(* Logix 5000 AddOnInstructionDefinition export Banner_S4B_PD_v5; software revision 33.00 *)

TYPE Banner_S4B_PDI_Host_Guest :
STRUCT
   Reduced_Resolution_Enabled : SINT;   // 0=false, 1=true
   Status : SINT;   // 0=clear, 1=weak beam, 2=blocked
   Indicator_State : SINT;   // 0=Enabled, 1=Override, 2=Dipswitch Disabled
   Measurement : INT;   // 0 to 180
   First_Channel_Blocked : INT;   // 0 to 180
   Number_Channels_Blocked : INT;   // 0 to 180
   Zone_1_Status : SINT;   // 0=clear, 1=weak beam, 2=blocked
   Zone_2_Status : SINT;   // 0=clear, 1=weak beam, 2=blocked
   Zone_3_Status : SINT;   // 0=clear, 1=weak beam, 2=blocked
END_STRUCT
END_TYPE

TYPE Banner_S4B_PDI_v5 :
STRUCT
   OSSD_Status : SINT;   // 0=Off, 1=On
   Weak_Beam_Flag : SINT;   // 0=Maintenance flag not active, 1=Maintenance flag active
   Cascaded_Units : SINT;   // 0=Standalone, 1=1 cascaded unit, 2=2 cascaded units, 3=3 cascaded units
   Configurable_IO_Pin_State : SINT;   // 0=Off, 1=On
   Fixed_Blanking_Enabled : SINT;   // 0=false, 1=true
   Vibration_Tolerance_Enabled : SINT;   // 0=false, 1=true
   Fault_Lockout : SINT;   // 0=false, 1=true
   Diagnostic_Error_Cocde : SINT;   // 0 to 255
   Host : Banner_S4B_PDI_Host_Guest;
   Guest_1 : Banner_S4B_PDI_Host_Guest;
   Guest_2 : Banner_S4B_PDI_Host_Guest;
   Guest_3 : Banner_S4B_PDI_Host_Guest;
END_STRUCT
END_TYPE

TYPE Banner_S4B_PDIO_v5 :   // UDT that records the converted prcoess data.
STRUCT
   PDI : Banner_S4B_PDI_v5;
   PDO : Banner_S4B_PDO_v5;
   PDO_DT : SINT[4];
   PDI_DT : SINT[20];
END_STRUCT
END_TYPE

TYPE Banner_S4B_PDO_v5 :
STRUCT
   Override_Indicator_State_Host : SINT;   // 0=Standard Operation, 1 to 9 = Override 1 to 9
   Override_Indicator_State_Guest_1 : SINT;   // 0=Standard Operation, 1 to 9 = Override 1 to 9
   Override_Indicator_State_Guest_2 : SINT;   // 0=Standard Operation, 1 to 9 = Override 1 to 9
   Override_Indicator_State_Guest_3 : SINT;   // 0=Standard Operation, 1 to 9 = Override 1 to 9
END_STRUCT
END_TYPE

ADD_ON_INSTRUCTION Banner_S4B_PD_v5   (* revision 5.0, vendor Banner Engineering *)
// Takes the raw SINT information and converts that data into actual information.
VAR_IN_OUT
   PD : Banner_S4B_PDIO_v5; {required}
END_VAR
VAR_INPUT
   Byte_Swap : BOOL; {required}
END_VAR
VAR
   PDO_Temp : SINT[4]; {access None}
   PDI_Temp : SINT[20]; {access None}
END_VAR

ROUTINE Logic   (* ladder *)
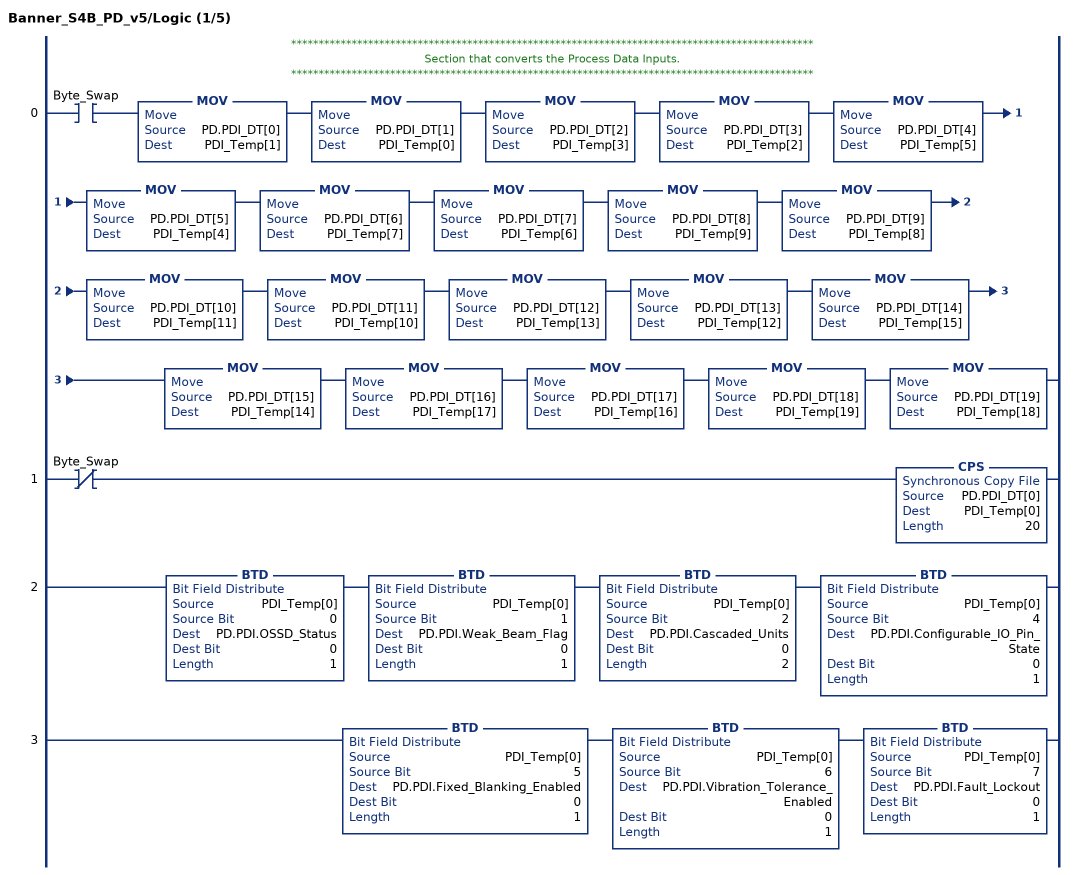
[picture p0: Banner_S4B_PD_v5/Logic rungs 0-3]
   // ***********************************************************************************************
   // Section that converts the Process Data Inputs.
   // ***********************************************************************************************
   0: XIC(Byte_Swap)MOV(PD.PDI_DT[0],PDI_Temp[1])MOV(PD.PDI_DT[1],PDI_Temp[0])MOV(PD.PDI_DT[2],PDI_Temp[3])MOV(PD.PDI_DT[3],PDI_Temp[2])MOV(PD.PDI_DT[4],PDI_Temp[5])MOV(PD.PDI_DT[5],PDI_Temp[4])MOV(PD.PDI_DT[6],PDI_Temp[7])MOV(PD.PDI_DT[7],PDI_Temp[6])MOV(PD.PDI_DT[8],PDI_Temp[9])MOV(PD.PDI_DT[9],PDI_Temp[8])MOV(PD.PDI_DT[10],PDI_Temp[11])MOV(PD.PDI_DT[11],PDI_Temp[10])MOV(PD.PDI_DT[12],PDI_Temp[13])MOV(PD.PDI_DT[13],PDI_Temp[12])MOV(PD.PDI_DT[14],PDI_Temp[15])MOV(PD.PDI_DT[15],PDI_Temp[14])MOV(PD.PDI_DT[16],PDI_Temp[17])MOV(PD.PDI_DT[17],PDI_Temp[16])MOV(PD.PDI_DT[18],PDI_Temp[19])MOV(PD.PDI_DT[19],PDI_Temp[18]);
   1: XIO(Byte_Swap)CPS(PD.PDI_DT[0],PDI_Temp[0],20);
   2: BTD(PDI_Temp[0],0,PD.PDI.OSSD_Status,0,1)BTD(PDI_Temp[0],1,PD.PDI.Weak_Beam_Flag,0,1)BTD(PDI_Temp[0],2,PD.PDI.Cascaded_Units,0,2)BTD(PDI_Temp[0],4,PD.PDI.Configurable_IO_Pin_State,0,1);
   3: BTD(PDI_Temp[0],5,PD.PDI.Fixed_Blanking_Enabled,0,1)BTD(PDI_Temp[0],6,PD.PDI.Vibration_Tolerance_Enabled,0,1)BTD(PDI_Temp[0],7,PD.PDI.Fault_Lockout,0,1);
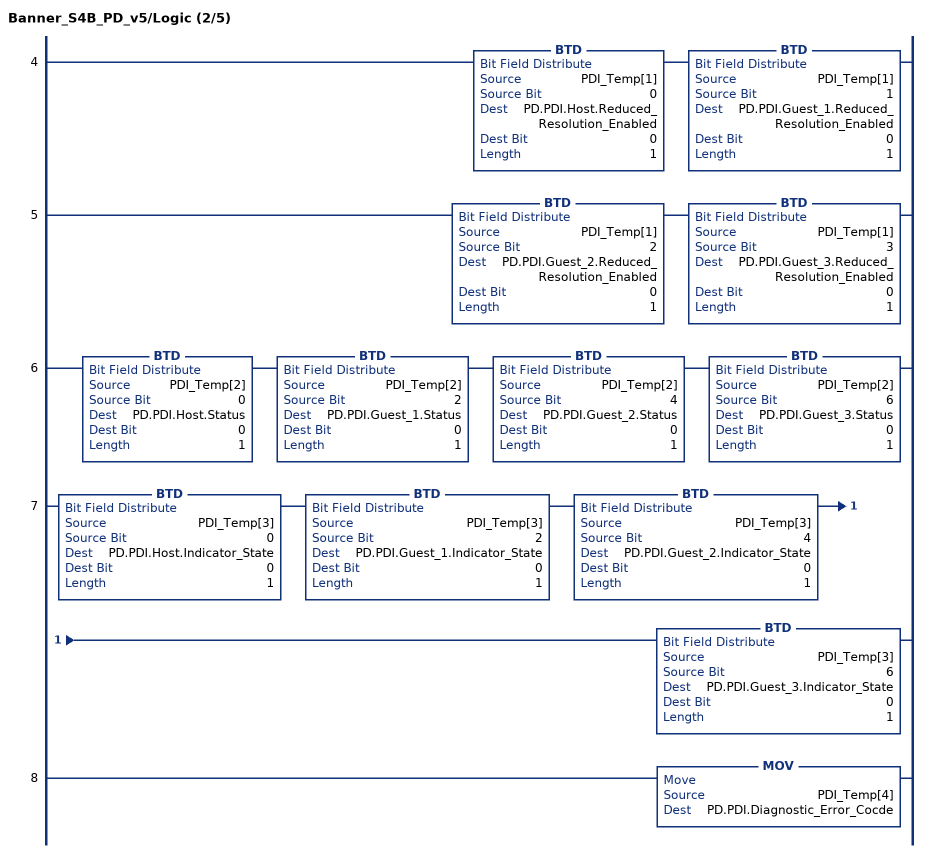
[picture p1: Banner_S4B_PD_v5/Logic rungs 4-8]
   4: BTD(PDI_Temp[1],0,PD.PDI.Host.Reduced_Resolution_Enabled,0,1)BTD(PDI_Temp[1],1,PD.PDI.Guest_1.Reduced_Resolution_Enabled,0,1);
   5: BTD(PDI_Temp[1],2,PD.PDI.Guest_2.Reduced_Resolution_Enabled,0,1)BTD(PDI_Temp[1],3,PD.PDI.Guest_3.Reduced_Resolution_Enabled,0,1);
   6: BTD(PDI_Temp[2],0,PD.PDI.Host.Status,0,1)BTD(PDI_Temp[2],2,PD.PDI.Guest_1.Status,0,1)BTD(PDI_Temp[2],4,PD.PDI.Guest_2.Status,0,1)BTD(PDI_Temp[2],6,PD.PDI.Guest_3.Status,0,1);
   7: BTD(PDI_Temp[3],0,PD.PDI.Host.Indicator_State,0,1)BTD(PDI_Temp[3],2,PD.PDI.Guest_1.Indicator_State,0,1)BTD(PDI_Temp[3],4,PD.PDI.Guest_2.Indicator_State,0,1)BTD(PDI_Temp[3],6,PD.PDI.Guest_3.Indicator_State,0,1);
   8: MOV(PDI_Temp[4],PD.PDI.Diagnostic_Error_Cocde);
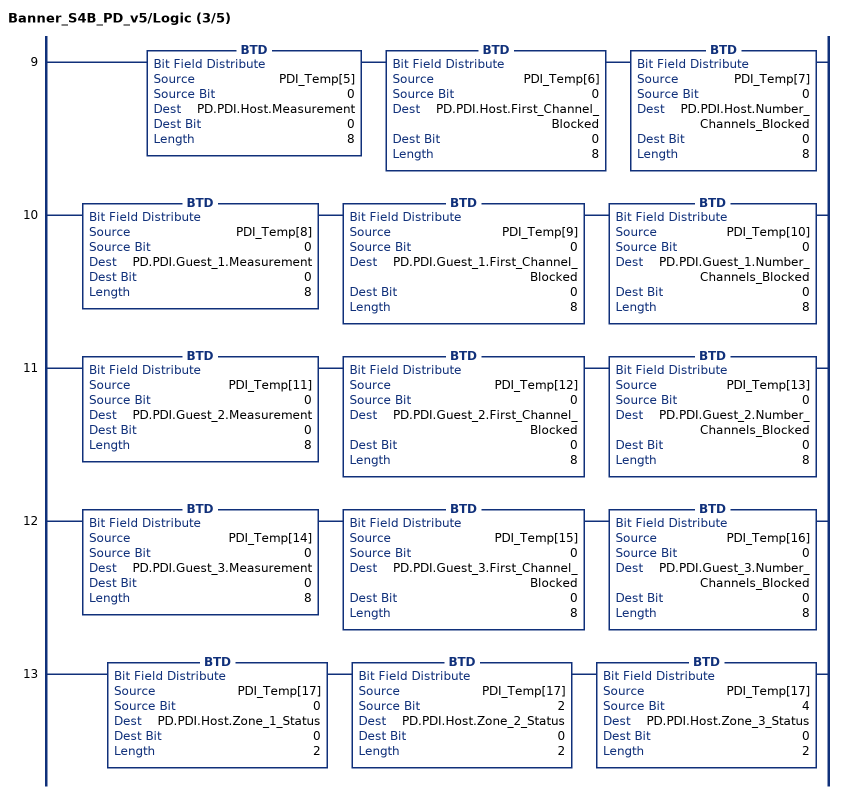
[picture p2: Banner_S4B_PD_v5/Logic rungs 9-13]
   9: BTD(PDI_Temp[5],0,PD.PDI.Host.Measurement,0,8)BTD(PDI_Temp[6],0,PD.PDI.Host.First_Channel_Blocked,0,8)BTD(PDI_Temp[7],0,PD.PDI.Host.Number_Channels_Blocked,0,8);
   10: BTD(PDI_Temp[8],0,PD.PDI.Guest_1.Measurement,0,8)BTD(PDI_Temp[9],0,PD.PDI.Guest_1.First_Channel_Blocked,0,8)BTD(PDI_Temp[10],0,PD.PDI.Guest_1.Number_Channels_Blocked,0,8);
   11: BTD(PDI_Temp[11],0,PD.PDI.Guest_2.Measurement,0,8)BTD(PDI_Temp[12],0,PD.PDI.Guest_2.First_Channel_Blocked,0,8)BTD(PDI_Temp[13],0,PD.PDI.Guest_2.Number_Channels_Blocked,0,8);
   12: BTD(PDI_Temp[14],0,PD.PDI.Guest_3.Measurement,0,8)BTD(PDI_Temp[15],0,PD.PDI.Guest_3.First_Channel_Blocked,0,8)BTD(PDI_Temp[16],0,PD.PDI.Guest_3.Number_Channels_Blocked,0,8);
   13: BTD(PDI_Temp[17],0,PD.PDI.Host.Zone_1_Status,0,2)BTD(PDI_Temp[17],2,PD.PDI.Host.Zone_2_Status,0,2)BTD(PDI_Temp[17],4,PD.PDI.Host.Zone_3_Status,0,2);
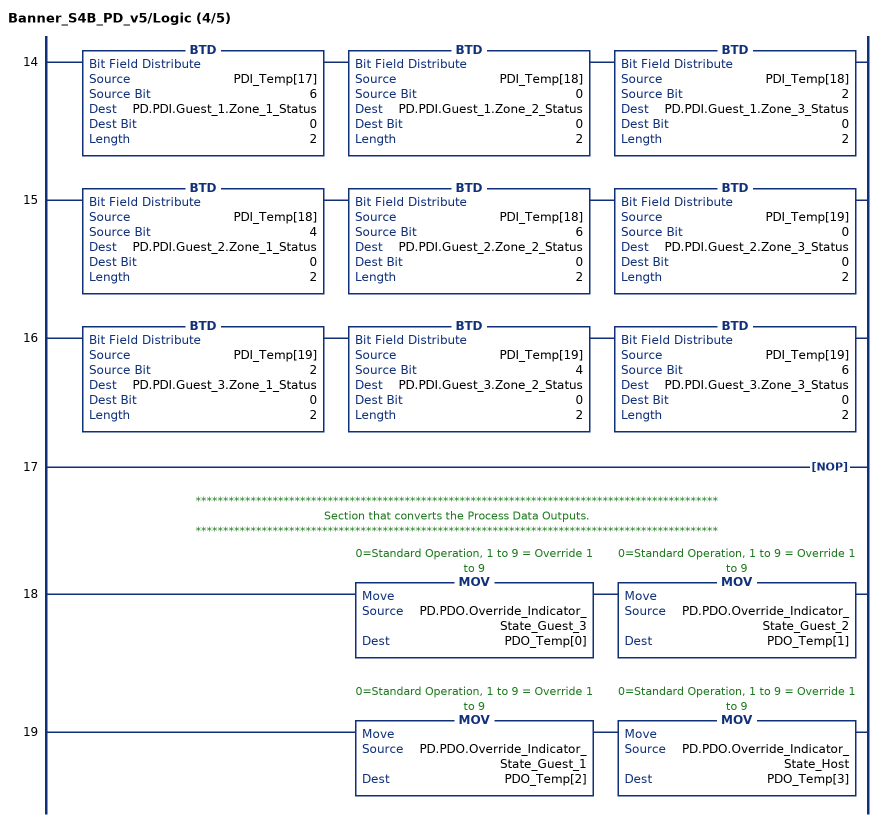
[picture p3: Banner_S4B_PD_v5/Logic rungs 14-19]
   14: BTD(PDI_Temp[17],6,PD.PDI.Guest_1.Zone_1_Status,0,2)BTD(PDI_Temp[18],0,PD.PDI.Guest_1.Zone_2_Status,0,2)BTD(PDI_Temp[18],2,PD.PDI.Guest_1.Zone_3_Status,0,2);
   15: BTD(PDI_Temp[18],4,PD.PDI.Guest_2.Zone_1_Status,0,2)BTD(PDI_Temp[18],6,PD.PDI.Guest_2.Zone_2_Status,0,2)BTD(PDI_Temp[19],0,PD.PDI.Guest_2.Zone_3_Status,0,2);
   16: BTD(PDI_Temp[19],2,PD.PDI.Guest_3.Zone_1_Status,0,2)BTD(PDI_Temp[19],4,PD.PDI.Guest_3.Zone_2_Status,0,2)BTD(PDI_Temp[19],6,PD.PDI.Guest_3.Zone_3_Status,0,2);
   17: NOP();
   // ***********************************************************************************************
   // Section that converts the Process Data Outputs.
   // ***********************************************************************************************
   18: MOV(PD.PDO.Override_Indicator_State_Guest_3,PDO_Temp[0])MOV(PD.PDO.Override_Indicator_State_Guest_2,PDO_Temp[1]);
   19: MOV(PD.PDO.Override_Indicator_State_Guest_1,PDO_Temp[2])MOV(PD.PDO.Override_Indicator_State_Host,PDO_Temp[3]);
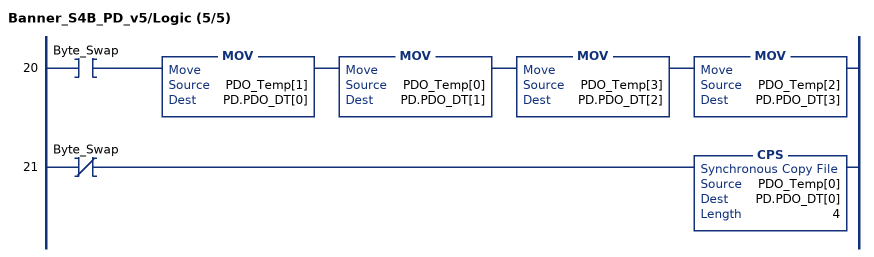
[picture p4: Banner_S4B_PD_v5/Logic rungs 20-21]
   20: XIC(Byte_Swap)MOV(PDO_Temp[1],PD.PDO_DT[0])MOV(PDO_Temp[0],PD.PDO_DT[1])MOV(PDO_Temp[3],PD.PDO_DT[2])MOV(PDO_Temp[2],PD.PDO_DT[3]);
   21: XIO(Byte_Swap)CPS(PDO_Temp[0],PD.PDO_DT[0],4);
END_ROUTINE
END_ADD_ON_INSTRUCTION
